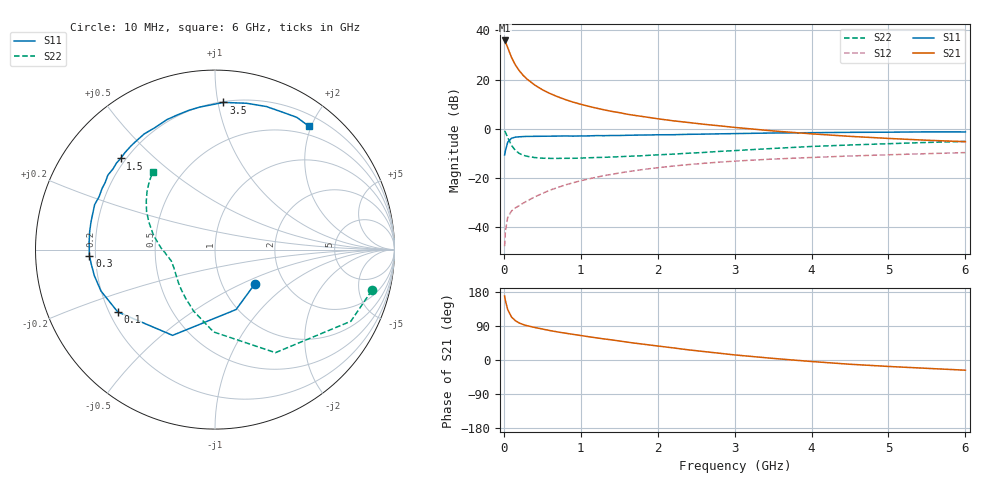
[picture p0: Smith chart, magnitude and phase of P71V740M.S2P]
! SIEMENS Small Signal Semiconductors
! BFP196
! Si NPN RF Bipolar Junction Transistor in SOT143
! VCE = 1.75 V  IC = 40 mA
! Common Emitter S-Parameters:  May  1996
# GHz  S  MA  R  50
!  f  S11  S21  S12  S22
! GHz  MAG  ANG  MAG  ANG  MAG  ANG  MAG  ANG
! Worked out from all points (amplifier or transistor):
!   36 points, 10 MHz to 6 GHz, reference 50 ohm
!   highest |S21| = 35.9 dB at 10 MHz (marker M1)
!   |S21| within 3 dB of that: start of sweep to 51.21 MHz
!   unconditionally stable (mu >= 1): 456.5 MHz to 4.348 GHz
!   at 250 MHz: K = 0.82, MSG = 26.0 dB, |S12| = -30.3 dB
!   at 1.4 GHz: K = 1.10, MAG = 10.9 dB, |S12| = -18.5 dB
!   at 6 GHz: K = 0.99, MSG = 2.2 dB, |S12| = -9.7 dB
!   S11 on the Smith chart (normalised r, x): 10 MHz: 1.42, -0.60; 100 MHz: 0.23, -0.28; 300 MHz: 0.18, -0.02; 1.5 GHz: 0.18, +0.39; 3.5 GHz: 0.21, +1.04; 6 GHz: 0.36, +1.96
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0.01  0.2932 -41.1  62.61 168.6  0.0041 80.2  0.9027 -14.6
0.02  0.354 -70.6  58.45 157.0  0.0081 71.3  0.8558 -27.8
0.05  0.533 -116.3  44.82 133.3  0.0157 54.8  0.6657 -59.6
0.1  0.6436 -147.3  28.25 113.4  0.0214 46.5  0.4587 -91.0
0.15  0.6761 -160.1  19.89 103.7  0.0246 46.6  0.363 -109.1
0.2  0.6877 -167.8  15.25 97.7  0.0274 49.2  0.3161 -121.3
0.25  0.6942 -173.3  12.26 93.7  0.0307 51.5  0.2904 -130.7
0.3  0.7005 -177.3  10.3 90.6  0.0339 53.3  0.2765 -137.0
0.4  0.7026 176.6  7.794 85.9  0.0411 57.2  0.26 -146.4
0.5  0.7056 171.7  6.246 81.8  0.0484 59.1  0.2527 -152.7
0.6  0.7079 167.3  5.216 77.7  0.0565 60.1  0.2503 -156.8
0.7  0.7108 162.9  4.486 74.0  0.0639 60.9  0.2501 -160.0
0.8  0.7159 159.5  3.927 70.8  0.0723 60.4  0.2512 -162.6
0.9  0.7097 155.6  3.488 67.7  0.0799 60.2  0.2512 -165.0
1.1  0.7168 148.6  2.874 61.5  0.0954 59.0  0.2573 -168.2
1.5  0.7307 136.0  2.135 50.3  0.126 54.3  0.2705 -173.5
2.2  0.7576 116.0  1.455 32.0  0.1746 44.7  0.3052 177.0
2.8  0.7895 100.7  1.151 17.9  0.2097 36.1  0.3469 167.8
3.5  0.8213 86.7  0.905 4.2  0.2424 26.3  0.3985 157.5
4.5  0.8469 70.3  0.702 -11.2  0.2799 14.4  0.4686 144.8
5.5  0.8664 58.3  0.585 -22.0  0.3122 3.6  0.5274 134.0
6  0.864 52.8  0.547 -26.9  0.3278 -2.1  0.5535 128.8
